(* Logix 5000 Rung export; software revision 16.04 *)

MODULES
   HARTTest : vendor None type None code None
END_MODULES

TYPE OutputData :
STRUCT
   Data : HART4Output;
END_STRUCT
END_TYPE

TYPE HART4Output :
STRUCT
   Channel_0 : REAL;
   Channel_1 : REAL;
   Channel_2 : REAL;
   Channel_3 : REAL;
END_STRUCT
END_TYPE

TYPE HARTDeviceStatus :
STRUCT
   LoopOpen : BOOL;
   CurrentUnderrange : BOOL;
   CurrentOverrange : BOOL;
   LoopShorted : BOOL;
   CalibrationBusy : BOOL;
   CalibrationFaulted : BOOL;
   HARTCommsFault : BOOL;
   RelayMessagesInhibited : BOOL;
END_STRUCT
END_TYPE

TYPE HARTStatus :
STRUCT
   ParityError : BOOL;
   OverrunError : BOOL;
   FramingError : BOOL;
   ChecksumError : BOOL;
   RxBufferOverflow : BOOL;
   ValueTooLarge : BOOL;
   ValueTooSmall : BOOL;
   NotEnoughBytesInCommand : BOOL;
   TransmitterSpecificCmdError : BOOL;
   InWriteProtectMode : BOOL;
   UpdateFailed : BOOL;
   AppliedProcessTooHigh : BOOL;
   AppliedProcessTooLow : BOOL;
   InMultidropMode : BOOL;
   InvalidUnitCode : BOOL;
   BothRangeValuesOutOfLimits : BOOL;
   PushedUpperRangeValueOverLimit : BOOL;
   AccessRestricted : BOOL;
   DeviceBusy : BOOL;
   CommandNotImplemented : BOOL;
   DeviceMalfunction : BOOL;
   ConfigurationChanged : BOOL;
   Coldstart : BOOL;
   MoreStatusAvailable : BOOL;
   LoopCurrentFixed : BOOL;
   LoopCurrentSaturated : BOOL;
   NonPrimaryVariableOutOFLimits : BOOL;
   PrimaryVariableOutOfLimites : BOOL;
END_STRUCT
END_TYPE

TYPE InputData :
STRUCT
   Data : HART4Input;
END_STRUCT
END_TYPE

TYPE HARTMessageRequest :
STRUCT
   Length : INT;
   StartCharacter : SINT;   // (0x82 for Long Address)
   AddressByte0 : SINT;   // (0x80 + Manufacturer ID)
   AddressByte1 : SINT;   // (Device Type Code)
   AddressByte2 : SINT;   // (Device ID Byte 0)
   AddressByte3 : SINT;   // (Device ID Byte 1)
   AddressByte4 : SINT;   // (Device ID Byte 2)
   CommandData : SINT[40];
END_STRUCT
END_TYPE

TYPE HARTModuleStatus :
STRUCT
   ConfigurationValid : BOOL;
   Channel0Enabled : BOOL;
   Channel1Enabled : BOOL;
   Channel2Enabled : BOOL;
   Channel3Enabled : BOOL;
   Channel0HARTEnabled : BOOL;
   Channel1HARTEnabled : BOOL;
   Channel2HARTEnabled : BOOL;
   Channel3HARTEnabled : BOOL;
END_STRUCT
END_TYPE

TYPE ProsoftSTRING16 :   // string type
STRUCT
   LEN : DINT;
   DATA : SINT[16];
END_STRUCT
END_TYPE

TYPE HARTMessageResponse :
STRUCT
   Status : INT;
   PacketLength : INT;
   StartCharacter : SINT;
   AddressByte0 : SINT;
   AddressByte1 : SINT;
   AddressByte2 : SINT;
   AddressByte3 : SINT;
   AddressByte4 : SINT;
   Command : SINT;
   ByteCount : SINT;
   Data : SINT[50];
END_STRUCT
END_TYPE

TYPE MessageControl :
STRUCT
   TriggerMessage : BOOL;
   MessageRequest : HARTMessageRequest;
   MessageResponse : HARTMessageResponse;
END_STRUCT
END_TYPE

TYPE HART_MODULEDEF :
STRUCT
   Input : InputData;   // Data Read from End Device
   Output : OutputData;   // Data Written to End Device
   Control : MessageControl;   // Message to be sent to End Device
END_STRUCT
END_TYPE

TYPE HART4Input :
STRUCT
   Instance : ProsoftSTRING16;
   ConfigurationStatus : HARTModuleStatus;
   Temperature : REAL;
   Ch0_ManufacturerID : SINT;
   Ch0_ManufacturerDeviceType : SINT;
   Ch0_DeviceID : DINT;
   Ch0_Tag : ProsoftSTRING8;
   Ch0_Descriptor : ProsoftSTRING16;
   Ch0_DeviceStatus : HARTDeviceStatus;
   Ch0_HARTStatus : HARTStatus;
   Ch0_RawCurrent : REAL;
   Ch0_ScaledValue : REAL;
   Ch0_DigitialCurrent : REAL;
   Ch0_PV : REAL;
   Ch0_SV : REAL;
   Ch0_TV : REAL;
   Ch0_FV : REAL;
   Ch0_PVUnitCode : SINT;
   Ch0_SVUnitCode : SINT;
   Ch0_TVUnitCode : SINT;
   Ch0_FVUnitCode : SINT;
   Ch0_Diagnostics : HARTDiagnostics;
   Ch1_ManufacturerID : SINT;
   Ch1_ManufacturerDeviceType : SINT;
   Ch1_DeviceID : DINT;
   Ch1_Tag : ProsoftSTRING8;
   Ch1_Descriptor : ProsoftSTRING16;
   Ch1_DeviceStatus : HARTDeviceStatus;
   Ch1_HARTStatus : HARTStatus;
   Ch1_RawCurrent : REAL;
   Ch1_ScaledValue : REAL;
   Ch1_DigitialCurrent : REAL;
   Ch1_PV : REAL;
   Ch1_SV : REAL;
   Ch1_TV : REAL;
   Ch1_FV : REAL;
   Ch1_PVUnitCode : SINT;
   Ch1_SVUnitCode : SINT;
   Ch1_TVUnitCode : SINT;
   Ch1_FVUnitCode : SINT;
   Ch1_Diagnostics : HARTDiagnostics;
   Ch2_ManufacturerID : SINT;
   Ch2_ManufacturerDeviceType : SINT;
   Ch2_DeviceID : DINT;
   Ch2_Tag : ProsoftSTRING8;
   Ch2_Descriptor : ProsoftSTRING16;
   Ch2_DeviceStatus : HARTDeviceStatus;
   Ch2_HARTStatus : HARTStatus;
   Ch2_RawCurrent : REAL;
   Ch2_ScaledValue : REAL;
   Ch2_DigitialCurrent : REAL;
   Ch2_PV : REAL;
   Ch2_SV : REAL;
   Ch2_TV : REAL;
   Ch2_FV : REAL;
   Ch2_PVUnitCode : SINT;
   Ch2_SVUnitCode : SINT;
   Ch2_TVUnitCode : SINT;
   Ch2_FVUnitCode : SINT;
   Ch2_Diagnostics : HARTDiagnostics;
   Ch3_ManufacturerID : SINT;
   Ch3_ManufacturerDeviceType : SINT;
   Ch3_DeviceID : DINT;
   Ch3_Tag : ProsoftSTRING8;
   Ch3_Descriptor : ProsoftSTRING16;
   Ch3_DeviceStatus : HARTDeviceStatus;
   Ch3_HARTStatus : HARTStatus;
   Ch3_RawCurrent : REAL;
   Ch3_ScaledValue : REAL;
   Ch3_DigitialCurrent : REAL;
   Ch3_PV : REAL;
   Ch3_SV : REAL;
   Ch3_TV : REAL;
   Ch3_FV : REAL;
   Ch3_PVUnitCode : SINT;
   Ch3_SVUnitCode : SINT;
   Ch3_TVUnitCode : SINT;
   Ch3_FVUnitCode : SINT;
   Ch3_Diagnostics : HARTDiagnostics;
END_STRUCT
END_TYPE

TYPE ProsoftSTRING8 :   // string type
STRUCT
   LEN : DINT;
   DATA : SINT[8];
END_STRUCT
END_TYPE

TYPE HARTDiagnostics :
STRUCT
   DeviceSpecificStatus0_0 : SINT;
   DeviceSpecificStatus0_1 : SINT;
   DeviceSpecificStatus0_2 : SINT;
   DeviceSpecificStatus0_3 : SINT;
   DeviceSpecificStatus0_4 : SINT;
   DeviceSpecificStatus0_5 : SINT;
   Reserved0 : SINT;
   Reserved1 : SINT;
   OperationMode_0 : SINT;
   OperationMode_1 : SINT;
   Reserved2 : SINT;
   Reserved3 : SINT;
   StandardizedStatus0 : SINT;
   StandardizedStatus1 : SINT;
   AnalogChannelSaturated : SINT;
   StandardizedStatus2 : SINT;
   StandardizedStatus3 : SINT;
   AnalogChannelFixed : SINT;
   DeviceSpecific1_0 : SINT;
   DeviceSpecific1_1 : SINT;
   DeviceSpecific1_2 : SINT;
   DeviceSpecific1_3 : SINT;
   DeviceSpecific1_4 : SINT;
   DeviceSpecific1_5 : SINT;
   DeviceSpecific1_6 : SINT;
   DeviceSpecific1_7 : SINT;
   DeviceSpecific1_8 : SINT;
   DeviceSpecific1_9 : SINT;
   DeviceSpecific1_10 : SINT;
END_STRUCT
END_TYPE

ADD_ON_INSTRUCTION PLX51HART4AOI   (* revision 1.0, vendor ProSoft Technology Inc. *)
// Add-On - PLX51-HART-4O Module
// Revision note:
// v1.00. Initial Release
VAR_IN_OUT
   Connection_Input : DINT[119]; {required}   // Input parameters.
   Connection_Output : DINT[4]; {required}   // Output parameters.
   PLX51HART : HART_MODULEDEF; {required}
        ._UTIL.PASSTHRU.MBMSG[0]   // Modbus reserved. Always 0.
        ._UTIL.PASSTHRU.MBMSG[3]   // Modbus Function Code received.
        ._UTIL.PASSTHRU.MBOFFSET   // Starting Address for Modbus data set.
        .DATA.READDATA[0]   // Reads the RadData array size.
   HARTMessage : MESSAGE; {required}
END_VAR

ROUTINE Logic   (* ladder *)
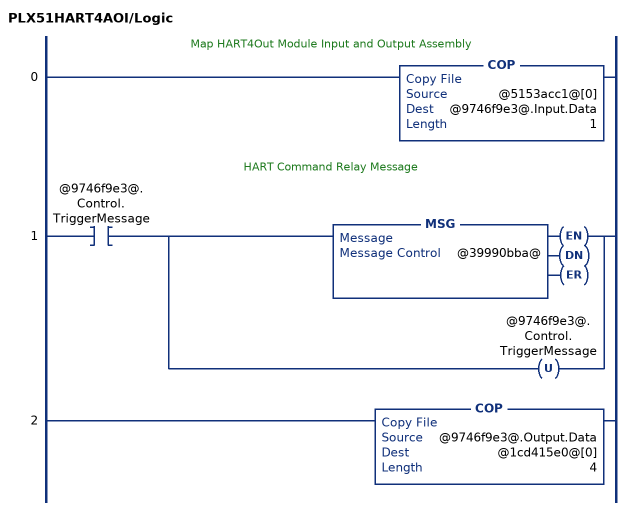
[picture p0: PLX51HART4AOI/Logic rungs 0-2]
   // Map HART4Out Module Input and Output Assembly
   0: COP(@5153acc1@[0],@9746f9e3@.Input.Data,1);
   // HART Command Relay Message
   1: XIC(@9746f9e3@.Control.TriggerMessage)[MSG(@39990bba@) ,OTU(@9746f9e3@.Control.TriggerMessage) ];
   2: COP(@9746f9e3@.Output.Data,@1cd415e0@[0],4);
END_ROUTINE
END_ADD_ON_INSTRUCTION

VAR_GLOBAL   (* controller tags *)
   HARTMessage : MESSAGE;
        MessageParameters(MessageType := CIP Generic, RequestedLength := 48, ConnectedFlag := 2, ConnectionPath := ENT2T, ServiceCode := 16#0079, ObjectType := 16#040f, TargetObject := 1, LocalElement := PLX51HART4O.Control.MessageRequest, DestinationTag := PLX51HART4O.Control.MessageResponse)
   HARTTest:O : AB:ETHERNET_MODULE_DINT_16Bytes:O:0;
   PLX51HART_AOI : PLX51HART4AOI;
   PLX51HART4O : HART_MODULEDEF;
   HARTTest:I : AB:ETHERNET_MODULE_DINT_476Bytes:I:0;
END_VAR

PROGRAM MainProgram

ROUTINE MainRoutine   (* ladder *)
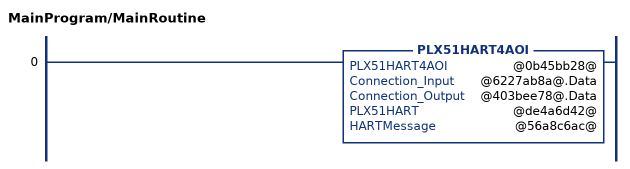
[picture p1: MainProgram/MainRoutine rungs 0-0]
   0: PLX51HART4AOI(@0b45bb28@,@6227ab8a@.Data,@403bee78@.Data,@de4a6d42@,@56a8c6ac@);
END_ROUTINE
END_PROGRAM
